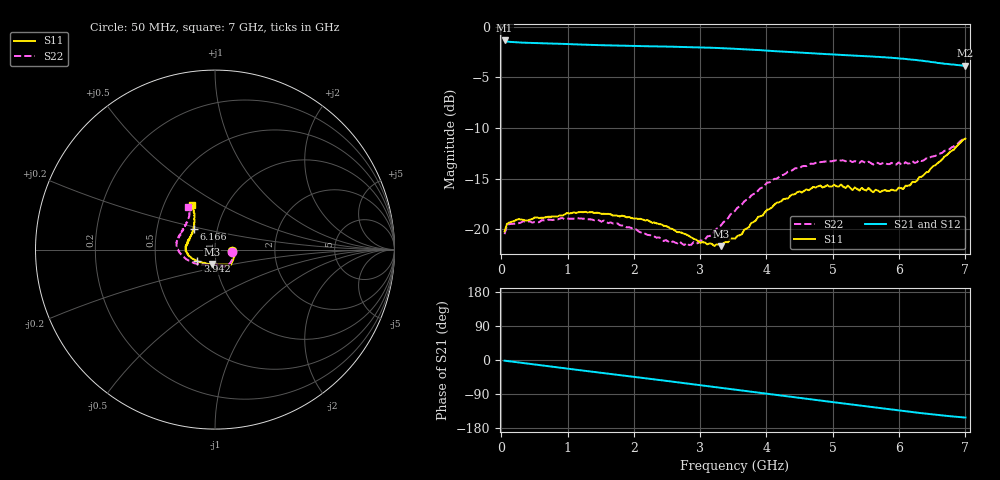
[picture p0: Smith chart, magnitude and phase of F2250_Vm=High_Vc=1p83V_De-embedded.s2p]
! Integrated Device Technology
! Corporate Headquarters
! 6024 Silver Creek Valley Road
! San Jose, CA 95138  USA
! Phone:  1-408-284-8200
! Toll Free:  1-800-223-1366
! Webpage:  http://www.idt.com/
! Timing and RF Division
! 515 Groton Road, Suite 102
! Westford, MA 01886-6024
! Device:  F2250
! Description: Voltage Variable RF Attenuator
! Frequency:  50.0 -  6000.00 MHz
! Package:  3x3 mm Thin QFN Plastic Package: 16 pin
! Ports:  2 RF, 3 DC
!  Pin  1  = GND
!  Pin  2  = NC
!  Pin  3  = RF1  = Port 1
!  Pin  4  = NC
!  Pin  5  = GND
!  Pin  6  = GND
!  Pin  7  = GND
!  Pin  8  = GND
!  Pin  9  = NC
!  Pin 10  = RF2  = Port 2
!  Pin 11  = NC
!  Pin 12  = GND
!  Pin 13  = GND
!  Pin 14  = VCNTRL
!  Pin 15  = VDD
!  Pin 16  = VMODE
! Vcntrl:  1.830 Volts
! Vmode:  +3.300 Volts
! Vdd:  +3.30  Volts
! Current:  1.324 mA
! Data:  The device was measured on a the F2250 evaluation board which has
!  individual transmission lines to the RF pins.  Data was collected
!  using a calibrated network analyzer.  The evaluation board was
!  de-embedded using a TRL calibration technique.
!  The reference plane is the edge of the package pin.
! Misc:  SN 10
!  Action Tracker AT0258
! Date Measured:  2014-11-26
! Date:  2015-10-15  MJV
! Note:
!  Integrated Device Technology supplies this data as a sample of measured
!  data at the package pin for this product.  Your particular data for this
!  product may vary.
!  Data was taken at 25 degrees C.
!  Integrated Device Technology reserves the right to change this data at anytime.
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# GHz S dB R 50
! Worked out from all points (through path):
!   201 points, 50 MHz to 7 GHz, reference 50 ohm
!   highest |S21| = -1.36 dB at 50 MHz (marker M1); lowest = -3.9 dB at 7 GHz (marker M2)
!   group delay of S21, straight-line fit = 61.1 ps
!   lowest |S11| = -21.7 dB at 3.317 GHz (marker M3), VSWR 1.18, Z = 47.7 - j7.75 ohm
!   |S11| at or under -10 dB: start of sweep to end of sweep
!   |S22| runs from -21.6 to -11.0 dB; largest |S21 - S12| = 0.002
!   S11 on the Smith chart (normalised r, x): 50 MHz: 1.21, -0.02; 3.942 GHz: 0.81, -0.10; 6.166 GHz: 0.77, +0.18; 7 GHz: 0.69, +0.37
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0.05  -20.22 -5.6  -1.36 -1.8  -1.36 -1.8  -20.49 -6.9
0.08475  -19.48 -5.5  -1.46 -2.5  -1.46 -2.5  -19.67 -6.4
0.1195  -19.34 -6.2  -1.50 -3.3  -1.50 -3.3  -19.49 -6.5
0.328  -19.07 -12.8  -1.58 -7.9  -1.58 -7.9  -19.22 -14.8
1.2315  -18.32 -42.4  -1.77 -27.9  -1.77 -27.9  -18.97 -51.8
1.75275  -18.67 -49.4  -1.87 -39.1  -1.87 -39.1  -19.42 -62.1
2.37825  -19.49 -52.4  -1.96 -52.6  -1.96 -52.6  -20.80 -72.1
2.552  -19.94 -55.8  -1.97 -56.5  -1.98 -56.5  -21.38 -78.6
2.86475  -20.80 -66.0  -2.02 -63.4  -2.02 -63.5  -21.54 -94.8
3.07325  -21.32 -79.4  -2.06 -68.1  -2.06 -68.2  -21.01 -109.8
3.3165  -21.68 -101.9  -2.11 -73.7  -2.12 -73.7  -19.60 -127.0
3.525  -20.94 -119.8  -2.18 -78.4  -2.19 -78.4  -18.20 -139.0
3.942  -18.66 -147.7  -2.33 -87.8  -2.34 -87.8  -15.87 -158.4
4.1505  -17.39 -157.0  -2.43 -92.4  -2.43 -92.5  -15.02 -166.7
4.4285  -16.54 -166.7  -2.53 -98.6  -2.54 -98.6  -13.99 -175.3
4.7065  -15.82 -175.3  -2.63 -104.7  -2.63 -104.7  -13.55 178.1
5.1235  -15.58 174.0  -2.78 -113.9  -2.78 -113.9  -13.21 168.4
5.29725  -16.13 168.3  -2.84 -117.6  -2.84 -117.7  -13.38 165.0
5.85325  -16.22 148.8  -3.06 -129.8  -3.06 -129.9  -13.58 150.5
6.166  -15.67 136.1  -3.23 -136.6  -3.23 -136.7  -13.50 141.7
6.54825  -13.68 124.2  -3.53 -144.5  -3.54 -144.6  -12.77 129.4
7  -11.05 117.6  -3.86 -151.9  -3.87 -152.0  -10.98 122.6
